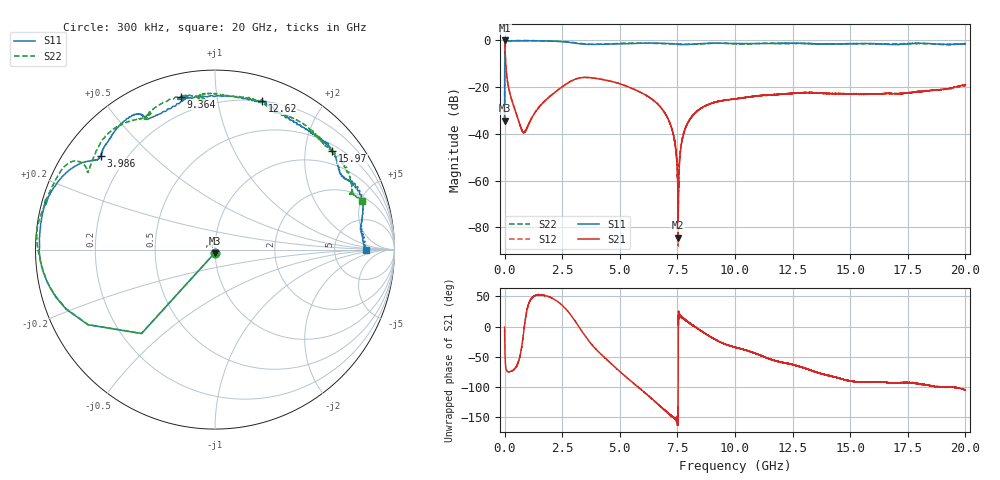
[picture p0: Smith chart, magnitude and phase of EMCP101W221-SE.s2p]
!EMCP101W221
!Johanson Technology Inc.
!www.johansontechnology.com
!Test Board Conditions:
!Substrate Type  RO4350B
!Substrate Thickness  10 mil
!Substrate Dk  3.66
!TL Type: GCPW
!TL Trace Width  20 mil
!TL Gap  10 mil
!PART MODE SINGLE ENDED (AKA BYPASS)
!DUT TOPOLOGY	SERIES-SHUNT
# MHz S  dB  R 50
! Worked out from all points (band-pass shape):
!   20001 points, 300 kHz to 20 GHz, reference 50 ohm
!   highest |S21| = -0.01 dB at 300 kHz (marker M1); lowest = -84.5 dB at 7.533 GHz (marker M2)
!   |S21| within 3 dB of the highest: start of sweep to 15.27 MHz
!   lowest |S11| = -34.4 dB at 300 kHz (marker M3), VSWR 1.04, Z = 49.8 - j1.9 ohm
!   |S11| at or under -10 dB: start of sweep to 5.35 MHz
!   |S22| runs from -34.6 to 0.0 dB; largest |S21 - S12| = 0.0064
!   S11 on the Smith chart (normalised r, x): 300 kHz: 1.00, -0.04; 3.986 GHz: 0.11, +0.35; 9.364 GHz: 0.11, +0.80; 12.62 GHz: 0.20, +1.34; 15.97 GHz: 0.66, +2.60; 20 GHz: 11, +0
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0.3  -34.37 -95.1  -0.01 -1.0  -0.02 -1.2  -34.56 -94.7
112.298  -0.31 -172.7  -16.60 -74.1  -16.55 -74.2  -0.33 -172.3
310.295  -0.19 179.7  -25.46 -73.9  -25.41 -74.1  -0.14 -179.1
825.288  -0.15 171.6  -39.32 -9.7  -39.38 -9.7  -0.03 173.8
1813.273  -0.24 162.5  -25.31 50.6  -25.21 50.7  -0.25 158.3
3334.25  -1.51 143.8  -15.92 -6.6  -15.93 -6.6  -1.34 147.3
3986.24  -1.68 140.7  -16.30 -38.4  -16.30 -38.3  -1.62 148.4
6667.2  -1.14 120.8  -27.46 -129.1  -27.42 -129.4  -1.32 123.7
7238.191  -1.41 118.3  -37.24 -148.2  -37.27 -147.8  -1.53 120.0
7365.19  -1.48 118.2  -42.20 -152.1  -42.30 -151.1  -1.54 119.4
7533.187  -1.76 117.1  -84.45 -47.7  -77.04 -74.2  -1.50 115.0
7600.186  -1.76 115.8  -50.96 19.2  -50.98 15.4  -1.52 115.3
7743.184  -1.76 113.2  -40.77 13.6  -40.88 14.2  -1.57 116.2
8018.18  -1.66 108.3  -34.14 5.7  -34.05 6.2  -1.65 117.5
9364.16  -1.18 102.6  -25.88 -25.7  -25.95 -24.9  -1.16 102.3
10000.15  -1.31 102.6  -25.03 -34.4  -24.88 -34.1  -1.44 94.4
11427.13  -1.31 75.2  -23.28 -52.6  -23.43 -52.1  -1.19 93.5
12621.11  -1.23 72.5  -22.52 -64.4  -22.47 -64.5  -1.28 80.1
13334.1  -1.44 67.2  -22.35 -73.0  -22.31 -73.4  -1.36 71.2
15972.06  -1.40 40.0  -23.00 -92.2  -22.91 -93.4  -1.45 48.5
16667.05  -1.72 32.6  -22.62 -93.0  -22.90 -93.0  -1.46 45.1
20000  -1.54 0.0  -18.99 -105.2  -19.24 -103.0  -1.27 18.4
